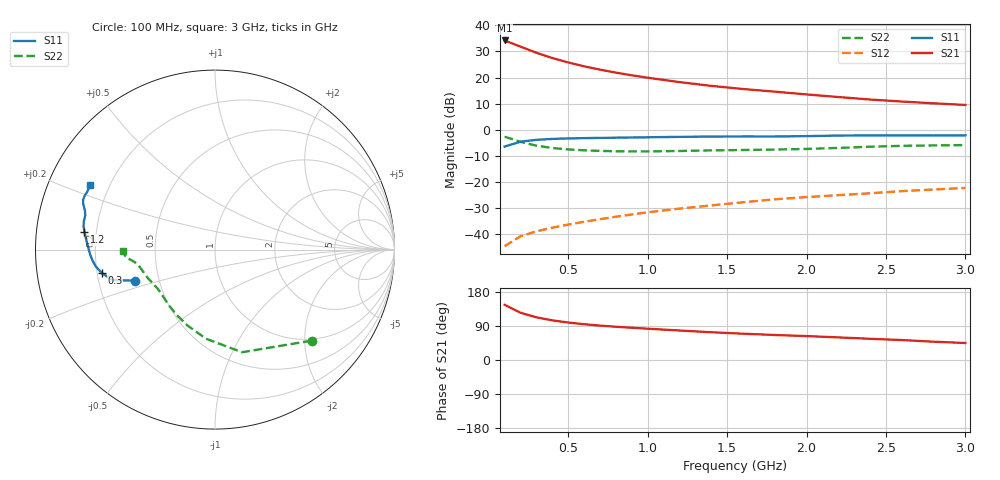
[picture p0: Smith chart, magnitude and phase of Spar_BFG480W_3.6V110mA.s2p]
! Filename: 3_6110BFG480.001
! Title: BFG480W
! Bias: Vce=3.6V; Ic=110mA
! Company: NXP Semiconductors NL
! User: Quality&Reliability T&D
! Measure time: 10 Nov 1999 / 12:01:12
#  MHz  S  MA  R 50
! Freq  S11  S21  S12  S22  :
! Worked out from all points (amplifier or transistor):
!   20 points, 100 MHz to 3 GHz, reference 50 ohm
!   highest |S21| = 34.2 dB at 100 MHz (marker M1)
!   |S21| within 3 dB of that: start of sweep to 227.5 MHz
!   unconditionally stable (mu >= 1): 660.9 MHz to end of sweep
!   at 400 MHz: K = 0.84, MSG = 32.4 dB, |S12| = -37.4 dB
!   at 1.2 GHz: K = 1.08, MAG = 22.4 dB, |S12| = -30.1 dB
!   at 3 GHz: K = 1.05, MAG = 14.5 dB, |S12| = -22.2 dB
!   S11 on the Smith chart (normalised r, x): 100 MHz: 0.36, -0.16; 300 MHz: 0.22, -0.10; 1.2 GHz: 0.15, +0.07; 3 GHz: 0.13, +0.24
100  0.4778 -158.8  51.16 145.7  0.005974 69.1  0.7396 -43.3
200  0.594 -163.4  39 124.7  0.009242 61.2  0.5915 -75.2
300  0.6444 -168.3  29.79 112.6  0.01147 60.5  0.499 -95.8
400  0.671 -172.0  23.62 104.6  0.01347 62.5  0.4498 -109.9
500  0.6849 -174.9  19.44 98.9  0.01544 64.9  0.4227 -120.1
600  0.6947 -177.3  16.4 94.4  0.0175 66.6  0.4065 -127.5
700  0.7015 -179.4  14.17 90.8  0.01956 68.7  0.3961 -133.3
800  0.7075 178.7  12.43 87.7  0.0218 70.3  0.3895 -138.1
900  0.7146 176.9  11.04 85.1  0.0241 71.9  0.3866 -142.3
1000  0.7209 175.2  9.924 82.6  0.02652 72.9  0.3869 -145.9
1200  0.734 172.3  8.186 77.9  0.03117 74.3  0.3946 -151.9
1400  0.7432 170.1  6.927 73.2  0.03589 75.1  0.4051 -156.2
1600  0.7476 167.8  6.042 69.4  0.04125 75.7  0.4117 -159.6
1800  0.7473 165.2  5.371 66.0  0.047 76.2  0.4195 -163.2
2000  0.7583 163.0  4.754 63.1  0.05179 76.6  0.4317 -167.5
2200  0.7768 161.0  4.241 59.6  0.05637 76.5  0.4512 -171.0
2400  0.7856 159.2  3.8 56.0  0.06128 75.9  0.4755 -173.3
2600  0.7854 157.6  3.474 52.7  0.06742 75.2  0.4945 -174.7
2800  0.781 155.3  3.219 48.3  0.07224 73.7  0.5039 -176.5
3000  0.7859 152.6  2.989 44.9  0.07757 72.9  0.5117 -179.3
